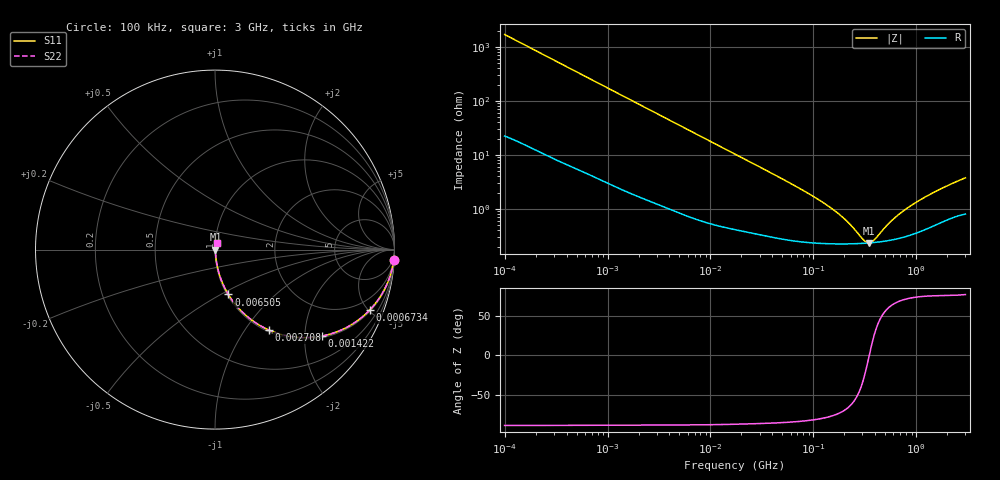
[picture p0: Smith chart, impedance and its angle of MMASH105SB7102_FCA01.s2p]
! MMASH105SB7102_FCA01  S-PARAMETER MODEL  ( Standard Model )
! Model Generated by TAIYO YUDEN Corporation (http://www.ty-top.com)
! Version 1.0
! TAIYO YUDEN Control No. 220601
! Copyright(c) 2019 TAIYO YUDEN CO.,LTD. All Rights Reserved.
! Product Description (link to TY-COMPAS)
! https://ds.yuden.co.jp/TYCOMPAS/or/detail?pn=MMASH105SB7102KFCA01&u=M
! Products Name : Multilayer Ceramic Capacitors
! Characteristics :
!  Capacitance : 1000 [pF] , Rated Voltage : 100 [V] , TCC : X7R
!  Case Size : 1.0 x 0.5 / 0.039 x 0.02 [mm/inch] , Thickness : 0.5 / 0.02 [mm/inch]
!  (Conditions: Temperature = 25 [degC] , DC Bias Voltage = 0 [V])
! External Node Assignments :
!  1  o---| |---o  2
! GND o---------o GND
! Frequency Range : 100kHz  -  3GHz  [ 401 STEP ]
# MHZ S RI R 50
! Freq[MHz].  S11 Real  S11 Imag  S21 Real  S21 Imag  S12 Real  S12 Imag  S22 Real  S22 Imag
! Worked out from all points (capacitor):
!   401 points, 100 kHz to 3 GHz, reference 50 ohm
!   read as one part in series: C = 937 pF near 105.3 kHz
!   lowest |Z| = 233 mohm at 344.3 MHz (marker M1)
!   series resonance near 348.9 MHz, so ESL is about 220 pH
!   S11 on the Smith chart (normalised r, x): 100 kHz: 1, -34; 673.4 kHz: 1.08, -5.12; 1.422 MHz: 1.04, -2.45; 2.708 MHz: 1.03, -1.29; 6.505 MHz: 1.01, -0.54; 3 GHz: 1.02, +0.07
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0.1  0.9958 -0.0587  0.00424 0.0587  0.00424 0.0587  0.9958 -0.0587
0.252895  0.9766 -0.1442  0.0234 0.1442  0.0234 0.1442  0.9766 -0.1442
0.562235  0.8999 -0.2922  0.1001 0.2922  0.1001 0.2922  0.8999 -0.2922
0.673391  0.8637 -0.3349  0.1363 0.3349  0.1363 0.3349  0.8637 -0.3349
0.965977  0.759 -0.4192  0.241 0.4192  0.241 0.4192  0.759 -0.4192
1.421866  0.5975 -0.4815  0.4025 0.4815  0.4025 0.4815  0.5975 -0.4815
1.937191  0.4487 -0.4879  0.5513 0.4879  0.5513 0.4879  0.4487 -0.4879
2.708188  0.2985 -0.4474  0.7015 0.4474  0.7015 0.4474  0.2985 -0.4474
3.161081  0.2401 -0.4166  0.7599 0.4166  0.7599 0.4166  0.2401 -0.4166
6.504802  0.0742 -0.2498  0.9258 0.2498  0.9258 0.2498  0.0742 -0.2498
17.7727  0.0139 -0.0985  0.9861 0.0985  0.9861 0.0985  0.0139 -0.0985
97.38194  0.00263 -0.0172  0.9974 0.0172  0.9974 0.0172  0.00263 -0.0172
180.7614  0.00228 -0.00738  0.9977 0.00738  0.9977 0.00738  0.00228 -0.00738
227.9507  0.00226 -0.00458  0.9977 0.00458  0.9977 0.00458  0.00226 -0.00458
310.5665  0.00229 -0.00122  0.9977 0.00122  0.9977 0.00122  0.00229 -0.00122
344.2911  0.00232 -0.000139  0.9977 0.000139  0.9977 0.000139  0.00232 -0.000139
391.6425  0.00237 0.0012  0.9976 -0.0012  0.9976 -0.0012  0.00237 0.0012
547.5153  0.00261 0.00482  0.9974 -0.00482  0.9974 -0.00482  0.00261 0.00482
745.9503  0.00302 0.00855  0.997 -0.00855  0.997 -0.00855  0.00302 0.00855
1097.999  0.00398 0.0141  0.996 -0.0141  0.996 -0.0141  0.00398 0.0141
1791.7  0.00619 0.0232  0.9938 -0.0232  0.9938 -0.0232  0.00619 0.0232
3000  0.00921 0.036  0.9908 -0.036  0.9908 -0.036  0.00921 0.036
